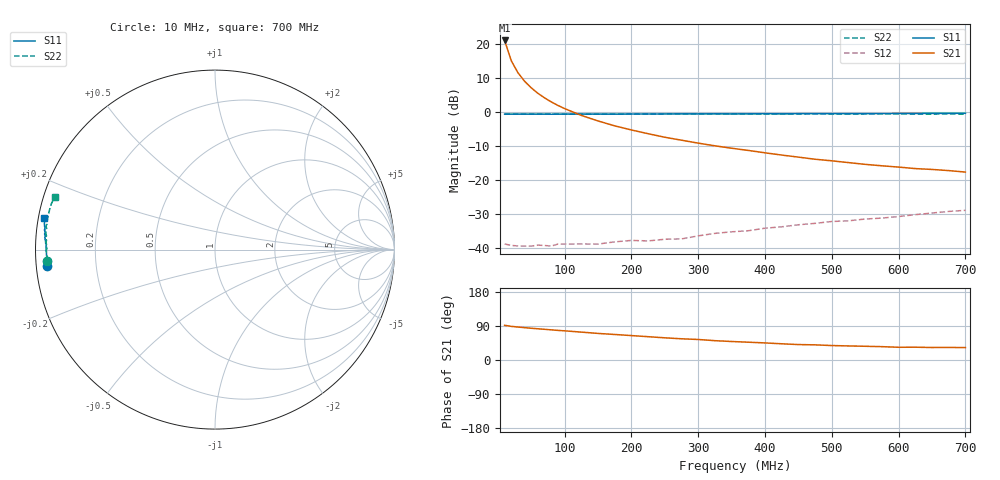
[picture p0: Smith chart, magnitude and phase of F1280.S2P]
! Date: Mon Aug 07 16:03:54 1995
# MHZ  S  MA  R  50.0000
!  POLYFET RF DEVICES
!  F1280
!  S PARAMETERS
!  VDS=12.5V, IDQ=1.20A
!FREQ  S11MAG S11ANG S21MAG S21ANG S12MAG S12ANG S22MAG S22ANG
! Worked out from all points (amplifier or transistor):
!   34 points, 10 MHz to 700 MHz, reference 50 ohm
!   highest |S21| = 21.1 dB at 10 MHz (marker M1)
!   |S21| within 3 dB of that: start of sweep to 15.02 MHz
!   unconditionally stable (mu >= 1): 175.7 MHz to end of sweep
!   at 60 MHz: K = 0.42, MSG = 22.3 dB, |S12| = -39.1 dB
!   at 300 MHz: K = 1.34, MAG = 10.2 dB, |S12| = -36.4 dB
!   at 700 MHz: K = 1.24, MAG = 2.7 dB, |S12| = -28.8 dB
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10  0.9406 -174.5  11.41 91.6  0.01155 7.4  0.9363 -176.3
20  0.9384 -177.4  5.735 88.7  0.01102 5.3  0.938 -178.4
30  0.9394 -178.4  3.817 87.0  0.0108 5.4  0.9395 -179.3
40  0.9393 -179.0  2.86 85.3  0.01073 8.1  0.9408 -179.9
50  0.9396 -179.5  2.287 83.8  0.01074 8.5  0.9393 179.7
60  0.9394 -179.7  1.9 82.4  0.01111 11.4  0.937 179.3
70  0.94 180.0  1.627 81.0  0.01098 13.6  0.9417 178.9
80  0.9369 179.8  1.42 79.6  0.01077 13.2  0.9414 178.6
90  0.9391 179.6  1.26 78.1  0.01152 17.7  0.9415 178.3
100  0.9412 179.4  1.133 77.0  0.01152 17.9  0.9404 177.9
125  0.9413 178.9  0.8997 73.5  0.01156 20.6  0.9415 177.4
150  0.9411 178.6  0.7459 70.1  0.01152 24.8  0.9404 176.8
175  0.9389 178.2  0.6316 67.4  0.01242 28.9  0.9448 176.1
200  0.9443 177.9  0.5498 64.4  0.01303 34.2  0.942 175.3
225  0.9446 177.4  0.4842 61.5  0.01283 39.2  0.9459 174.8
250  0.9463 176.9  0.4294 58.5  0.01356 40.1  0.9464 174.1
275  0.9492 176.6  0.3888 56.0  0.01373 45.5  0.9437 173.3
325  0.9512 175.9  0.3214 51.0  0.01656 48.6  0.9508 172.0
375  0.9504 175.2  0.2747 47.0  0.0181 52.5  0.9465 170.7
475  0.9547 173.4  0.2039 40.0  0.02325 58.8  0.9498 168.0
600  0.9616 171.3  0.1564 33.6  0.02929 61.0  0.9474 164.5
700  0.9676 169.6  0.1321 32.7  0.03614 60.3  0.9411 161.8
